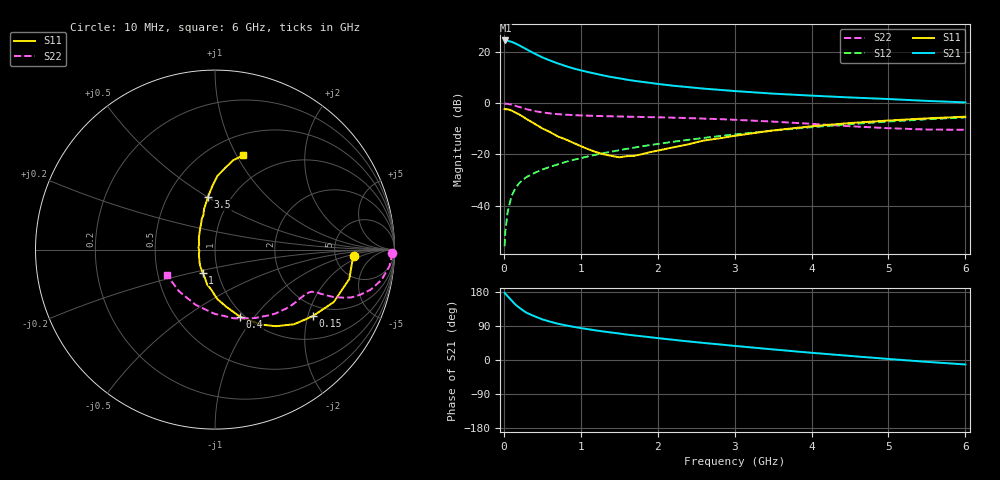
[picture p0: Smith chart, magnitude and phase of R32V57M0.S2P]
! SIEMENS Small Signal Semiconductors
! BFR181
! Si NPN RF Bipolar Junction Transistor in SOT23
! VCE = 2.5 V  IC = 7 mA
! Common Emitter S-Parameters:  May  1996
# GHz  S  MA  R  50
!  f  S11  S21  S12  S22
! GHz  MAG  ANG  MAG  ANG  MAG  ANG  MAG  ANG
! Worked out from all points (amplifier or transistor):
!   36 points, 10 MHz to 6 GHz, reference 50 ohm
!   highest |S21| = 24.6 dB at 20 MHz (marker M1)
!   |S21| within 3 dB of that: start of sweep to 266.6 MHz
!   unconditionally stable (mu >= 1): 896.2 MHz to 2.765 GHz
!   at 250 MHz: K = 0.52, MSG = 25.9 dB, |S12| = -29.9 dB
!   at 1.4 GHz: K = 1.06, MAG = 13.1 dB, |S12| = -18.9 dB
!   at 6 GHz: K = 0.85, MSG = 2.9 dB, |S12| = -5.5 dB
!   S11 on the Smith chart (normalised r, x): 10 MHz: 7.67, -1.41; 150 MHz: 1.64, -2.15; 400 MHz: 0.95, -0.85; 1 GHz: 0.84, -0.22; 3.5 GHz: 0.78, +0.50; 6 GHz: 0.71, +1.06
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0.01  0.776 -2.7  17 177.5  0.0016 90.4  0.9876 -1.1
0.02  0.7673 -5.2  17.01 174.9  0.0032 81.5  0.9853 -2.2
0.05  0.7659 -12.3  16.78 168.1  0.0075 79.9  0.9763 -5.5
0.1  0.7235 -23.8  15.96 157.3  0.0153 78.7  0.943 -10.3
0.15  0.6587 -34.3  14.9 146.3  0.0218 72.9  0.8951 -14.5
0.2  0.6063 -43.3  13.63 138.2  0.0274 70.7  0.8481 -17.2
0.25  0.5448 -51.6  12.42 130.6  0.0321 67.6  0.8056 -19.3
0.3  0.4873 -58.8  11.31 124.2  0.0365 67.2  0.7652 -20.5
0.4  0.3988 -69.6  9.424 115.3  0.0435 65.4  0.7059 -21.9
0.5  0.3236 -79.0  7.937 107.2  0.0505 65.4  0.6646 -22.4
0.6  0.2744 -87.6  6.896 101.2  0.0572 65.7  0.6348 -22.7
0.7  0.2253 -95.1  6.066 95.9  0.0637 66.3  0.614 -22.9
0.8  0.1976 -103.2  5.38 91.6  0.0711 66.1  0.5998 -23.2
1  0.1452 -118.3  4.422 84.3  0.0844 66.9  0.5798 -24.1
1.1  0.1259 -130.1  4.075 81.2  0.0919 67.3  0.5732 -24.8
1.3  0.1005 -150.6  3.496 75.2  0.1065 67.2  0.5617 -26.3
1.6  0.0925 173.0  2.901 67.0  0.1288 66.7  0.5488 -29.2
2.2  0.1373 127.8  2.213 53.4  0.1767 64.3  0.5242 -36.9
3.5  0.2953 97.6  1.548 27.9  0.2923 54.6  0.4387 -60.8
4.5  0.4113 88.1  1.303 10.8  0.3911 43.8  0.3565 -90.9
5.5  0.5081 78.5  1.116 -4.9  0.4874 30.9  0.3068 -130.8
6  0.5476 73.4  1.043 -11.8  0.5301 23.7  0.3036 -152.7
